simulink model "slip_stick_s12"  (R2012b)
settings: Solver=ode2  StartTime=0.0  StopTime=100  FixedStep=0.001  MaxStep=0.001  RelTol=1e-3
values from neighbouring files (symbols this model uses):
  FG = 500    [coulomb_1.m]    (also in coulomb_10.m = 10; coulomb_11.m = 10; coulomb_2.m; coulomb_3.m)
  FH = 12    [coulomb_10.m]    (also in coulomb_11.m; coulomb_3.m = 600; coulomb_4.m = 600; position_reg_1.m = 3.956)
  k = 10    [coulomb_10.m]    (also in coulomb_11.m; diff_filter_1.m = 250; diff_filter_2.m = 250; dry_friction_1.m = 2200)
  m = 400    [coulomb_1.m]    (also in coulomb_10.m = 10; coulomb_11.m = 10; coulomb_2.m; coulomb_3.m)
  sigma_0 = 5000    [position_reg_1.m]    (also in position_reg_2.m; slip_stick_21.m = 10000; slip_stick_s_12.m = 10000; tilger_gleitreib2.m = 1000)
  sigma_1 = sqrt(sigma_0)    [position_reg_1.m]    (also in position_reg_2.m; slip_stick_21.m = sqrt(1e5); slip_stick_s_12.m = sqrt(1e5); tilger_gleitreib2.m)
  sigma_2 = 0    [position_reg_1.m]    (also in position_reg_2.m; slip_stick_21.m; slip_stick_s_12.m; tilger_gleitreib2.m)
  vb = 0.1    [coulomb_10.m]    (also in coulomb_11.m; slip_stick_3.m; slip_stick_31.m; slip_stick_3_1.m)
  vs = 0.05    [position_reg_1.m]    (also in position_reg_2.m; slip_stick_21.m; slip_stick_3.m = 0.01; slip_stick_31.m)

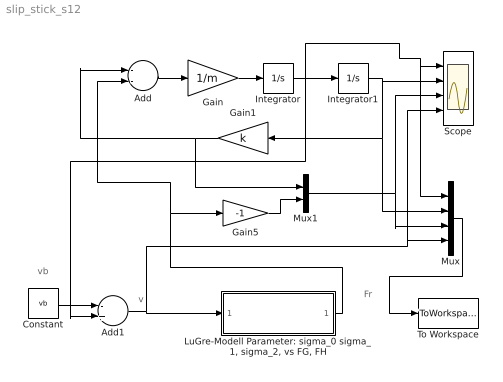
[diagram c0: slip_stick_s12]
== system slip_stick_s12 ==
  note: v
  note: vb
  note: Fr
  Add : Sum  Inputs=--
  Add1 : Sum  Inputs=-+
  Constant : Constant  Value=vb
  Gain : Gain  Gain=1/m
  Gain1 : Gain  Gain=k
  Gain5 : Gain  Gain=-1
  Integrator : Integrator
  Integrator1 : Integrator
  "LuGre-Modell Parameter: sigma_0 sigma_1, sigma_2, vs FG, FH" : Subsystem
  Mux : Mux
  Mux1 : Mux  Inputs=2
  Scope : Scope  NumInputPorts=4
  To Workspace : ToWorkspace  VariableName=y  SampleTime=-1  SaveFormat=Structure With Time
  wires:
  Add/1 -> Gain/1
  Gain/1 -> Integrator/1
  Integrator1/1 -> Mux/2, Gain1/1, Scope/2
  Constant/1 -> Add1/1
  Integrator/1 -> Add1/2, Integrator1/1, Mux/1, Scope/1
  "LuGre-Modell Parameter: sigma_0 sigma_1, sigma_2, vs FG, FH"/1(Fr) -> Add/2, Gain5/1
  Gain1/1 -> Mux1/1, Add/1
  Mux1/1 -> Mux/3, Scope/3
  Gain5/1 -> Mux1/2
  Add1/1 -> Mux/4, Scope/4, "LuGre-Modell Parameter: sigma_0 sigma_1, sigma_2, vs FG, FH"/1(v)
  Mux/1 -> To Workspace/1

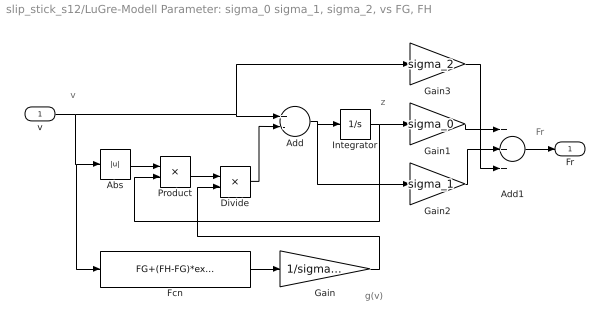
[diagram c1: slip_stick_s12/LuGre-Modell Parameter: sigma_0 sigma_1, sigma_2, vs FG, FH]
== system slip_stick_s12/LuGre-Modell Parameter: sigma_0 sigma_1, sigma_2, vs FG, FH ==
  note: z
  note: g(v)
  note: v
  note: Fr
  v : Inport
  Abs : Abs
  Add : Sum  Inputs=+-
  Add1 : Sum  Inputs=+++
  Divide : Product  Inputs=*/
  Fcn : Fcn  Expr=FG+(FH-FG)*exp(-(u/vs)^2)
  Gain : Gain  Gain=1/sigma_0
  Gain1 : Gain  Gain=sigma_0
  Gain2 : Gain  Gain=sigma_1
  Gain3 : Gain  Gain=sigma_2
  Integrator : Integrator
  Product : Product
  Fr : Outport
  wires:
  Product/1 -> Divide/1
  Gain/1 -> Divide/2
  Fcn/1 -> Gain/1
  Gain3/1 -> Add1/3
  Add1/1 -> Fr/1
  Gain1/1 -> Add1/1
  Divide/1 -> Add/2
  Abs/1 -> Product/1
  Gain2/1 -> Add1/2
  Add/1 -> Integrator/1, Gain2/1
  Integrator/1 -> Product/2, Gain1/1
  v/1 -> Abs/1, Fcn/1, Add/1, Gain3/1
